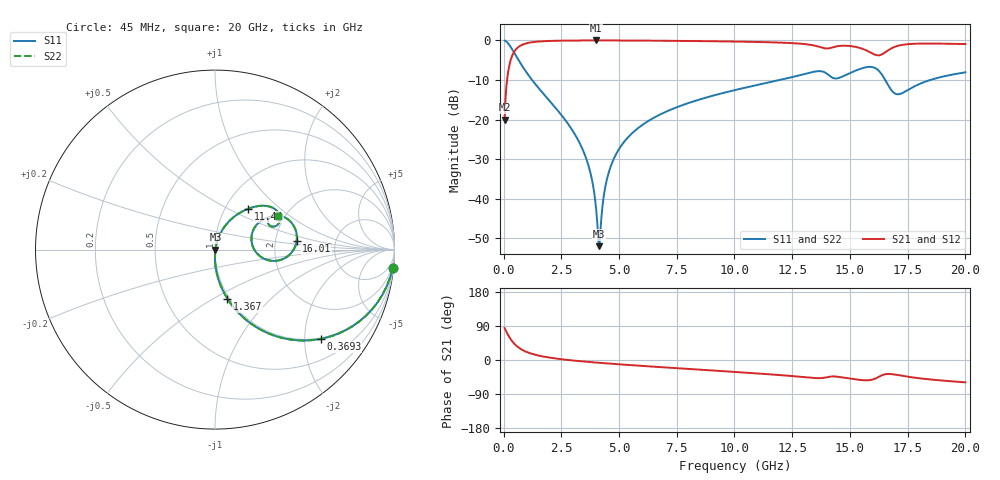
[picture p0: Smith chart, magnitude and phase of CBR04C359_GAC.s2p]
! S-parameter model data by Modelithics Inc.  support@modelithics.com 813-866-6335  Tampa FL USA
! S-Parameter data specifications:
! Substrate: 20-mil Rogers 4350B, substrate thickness, H=0.508mm, Dielectric constant, Er=3.75
! PCB Mounting Pad Footprint: Pad width, PadW=0.52mm , Pad length, PadL=0.52mm , Pad gap, PadG (edge-to-edge)=0.28mm , Reference planes=1.32mm apart
#  GHz  S  MA  R 50
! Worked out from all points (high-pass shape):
!   801 points, 45 MHz to 20 GHz, reference 50 ohm
!   highest |S21| = -0.02 dB at 4.011 GHz (marker M1); lowest = -20.1 dB at 45 MHz (marker M2)
!   |S21| within 3 dB of the highest: 445.5 MHz to 15.87 GHz (15.43 GHz wide, 189 % of centre); 16.53 GHz to end of sweep
!   lowest |S11| = -52.0 dB at 4.136 GHz (marker M3), VSWR 1.01, Z = 50.2 - j0.0444 ohm
!   |S11| at or under -10 dB: 1.234 GHz to 11.97 GHz (10.73 GHz wide, 163 % of centre); 16.53 GHz to 18.48 GHz (1.955 GHz wide, 11.2 % of centre)
!   |S22| runs from -52.0 to 0.0 dB; largest |S21 - S12| = 0
!   S11 on the Smith chart (normalised r, x): 45 MHz: 1, -20; 369.3 MHz: 0.97, -2.39; 1.367 GHz: 0.98, -0.58; 11.44 GHz: 1.27, +0.63; 16.01 GHz: 2.64, +0.31; 20 GHz: 1.84, +0.81
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0.045  0.9951 -5.8  0.0992 84.2  0.0992 84.2  0.9951 -5.8
0.219606  0.8986 -26.4  0.4384 63.6  0.4384 63.6  0.8986 -26.4
0.369269  0.7713 -40.1  0.6359 49.8  0.6359 49.8  0.7713 -40.1
0.768369  0.4932 -61.7  0.8689 28.2  0.8689 28.2  0.4932 -61.7
1.367019  0.2823 -75.8  0.9579 14.0  0.9579 14.0  0.2823 -75.8
3.387462  0.04431 -90.6  0.9966 -3.5  0.9966 -3.5  0.04431 -90.6
3.786563  0.01973 -88.7  0.9973 -5.6  0.9973 -5.6  0.01973 -88.7
4.011056  0.007308 -77.0  0.9974 -6.8  0.9974 -6.8  0.007308 -77.0
4.135775  0.002513 -10.1  0.9974 -7.4  0.9974 -7.4  0.002513 -10.1
4.460044  0.01681 72.1  0.9971 -8.9  0.9971 -8.9  0.01681 72.1
4.859144  0.03591 74.9  0.9965 -10.7  0.9965 -10.7  0.03591 74.9
5.582512  0.06785 73.7  0.9946 -13.9  0.9946 -13.9  0.06785 73.7
6.704981  0.1129 69.9  0.9901 -18.4  0.9901 -18.4  0.1129 69.9
10.0225  0.2356 57.2  0.9663 -31.5  0.9663 -31.5  0.2356 57.2
11.44429  0.2925 51.0  0.9477 -37.4  0.9477 -37.4  0.2925 51.0
13.36496  0.3968 36.0  0.8706 -47.0  0.8706 -47.0  0.3968 36.0
14.4126  0.3301 26.4  0.8382 -43.8  0.8382 -43.8  0.3301 26.4
15.31058  0.422 25.8  0.8193 -51.7  0.8193 -51.7  0.422 25.8
16.009  0.4571 5.8  0.6735 -51.1  0.6735 -51.1  0.4571 5.8
16.68248  0.2635 -9.5  0.7579 -36.7  0.7579 -36.7  0.2635 -9.5
17.13147  0.2092 13.4  0.8614 -40.3  0.8614 -40.3  0.2092 13.4
20  0.3946 28.0  0.8978 -59.0  0.8978 -59.0  0.3946 28.0
